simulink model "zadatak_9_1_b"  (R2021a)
settings: Solver=VariableStepAuto  StartTime=0.0  StopTime=2/50  RelTol=1e-3
libraries: spsGroundLib x4, spsVoltageMeasurementLib x2, spsACVoltageSourceLib x1, spsSeriesRLCLoadLib x1, spsThyristorLib x1, spspowerguiLib x1

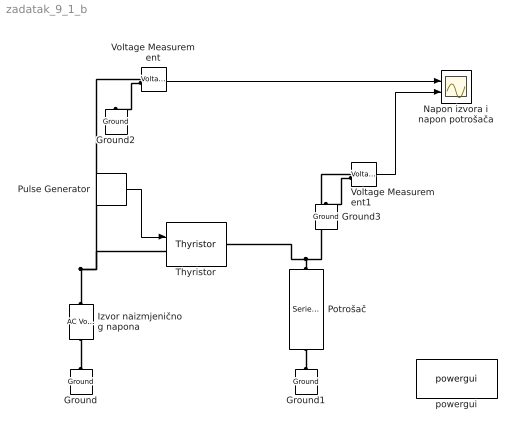
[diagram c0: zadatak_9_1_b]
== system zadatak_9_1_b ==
  Ground{,1..3} (4 alike) : spsGroundLib/Ground  LConnTagsString=a
  Izvor naizmjeničnog napona : spsACVoltageSourceLib/AC Voltage Source  Amplitude=220*sqrt(2)  Phase=0  Frequency=50  SampleTime=0  Measurements=None  BusType=swing  Pref=10e3  Qref=0  Qmin=-inf  Qmax=+inf
  Napon izvora i napon potrošača : Scope  NumInputPorts=2
  Potrošač : spsSeriesRLCLoadLib/Series RLC Load  LConnTagsString=a  RConnTagsString=__new0  NominalVoltage=220*sqrt(2)/2  NominalFrequency=50  ActivePower=1.5e3  InductivePower=0  CapacitivePower=0  Setx0=off  InitialVoltage=0  SetiL0=off  InitialCurrent=0  Measurements=None  LoadType=constant Z
  Pulse Generator : DiscretePulseGenerator  PulseType=Time based  Period=1/50  PulseWidth=5  PhaseDelay=30/360*1/50
  Thyristor : spsThyristorLib/Thyristor  Ron=0.001  Lon=0  Vf=0.8  IC=0  Rs=500  Cs=250e-9  Measurements=off
  Voltage Measurement : spsVoltageMeasurementLib/Voltage Measurement  PhasorSimulation=off  OutputType=Complex  PSBequivalent=0
  Voltage Measurement1 : spsVoltageMeasurementLib/Voltage Measurement  PhasorSimulation=off  OutputType=Complex  PSBequivalent=0
  powergui : spspowerguiLib/powergui  Priority=1  SimulationMode=Discrete  SampleTime=1e-6  frequency=60  Iterations=50  frequencyindice=50  Pbase=100e6  ErrMax=1e-4  UnitsV=kV  UnitsW=MW  buscounter=0  FunctionMessages=off  echomessages=off  EnableUseOfTLC=off  CurrentSourceSwitches=off  DisableSnubberDevices=off  DisableRonSwitches=off  DisableVfSwitches=off  DisplayEquations=off  AutomaticDiscreteSolvers=off  SolverType=Tustin/Backward Euler (TBE)  Interpol=off  ExternalGateDelay=off  methode=off  Ts=100  x0status=blocks  SPID=on  SwTol=0  HookPort=off  NonlinearTolerance=1e-4  nMaxIteration=100  ContinueOnMaxIteration=off  RestoreLinks=warning  ResistiveCurrentMeasurement=off  Frange=[0:2:500]  Ylog=off  Xlog=on  ShowGrid=off  save=off  variable=ZData  structure=0  ZoomFFT=off  StartTime=0.0  cycles=1  DisplayStyle=1  fundamental=60  FreqAxis=off  MaxFrequency=1000  frequencyindicesteady=1  RmsSteady=1  display=off
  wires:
  Voltage Measurement/1 -> Napon izvora i napon potrošača/1
  Voltage Measurement1/1 -> Napon izvora i napon potrošača/2
  Pulse Generator/1 -> Thyristor/1
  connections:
  Ground/LConn1 -- Izvor naizmjeničnog napona/LConn1
  Izvor naizmjeničnog napona/RConn1 -- Thyristor/LConn1 -- Voltage Measurement/LConn1
  Potrošač/LConn1 -- Thyristor/RConn1 -- Voltage Measurement1/LConn1
  Ground1/LConn1 -- Potrošač/RConn1
  Voltage Measurement/LConn2 -- Ground2/LConn1
  Voltage Measurement1/LConn2 -- Ground3/LConn1
